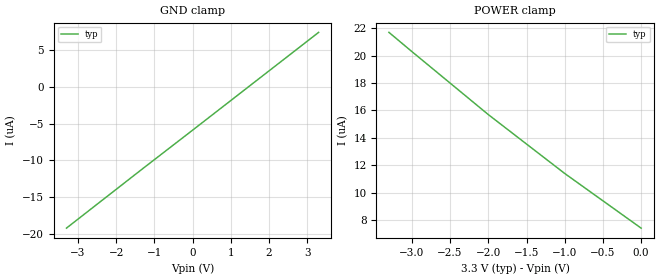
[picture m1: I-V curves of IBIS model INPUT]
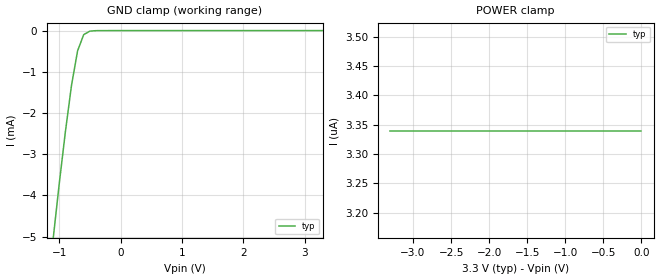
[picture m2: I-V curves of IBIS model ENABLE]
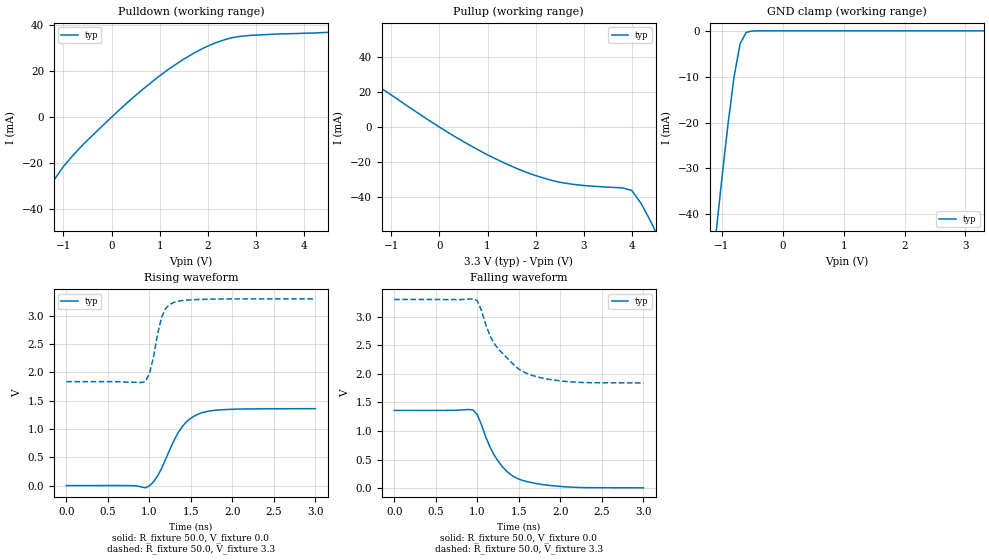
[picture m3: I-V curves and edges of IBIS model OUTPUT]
|   Texas Instruments Incorporated
|   Data Transmissions Products
|   IBIS Model for SN65LVDS348
|   16D SOIC Package
[IBIS Ver]   3.2
[Comment char]   |_char
[File name]   lvds348.ibs
[File Rev]   1.0
[Date]   23Aug01
[Source]   File originated at Texas Instruments Incorporated.
   Data Transmission Products Group. All data based on
   Bench Measurements.
[Notes]
[Disclaimer]
(C) Copyright Texas Instruments Incorporated 2001
   All rights reserved
  Texas Instruments Incorporated hereby grants the user of this IBIS
model a non-exclusive, nontransferable license to use this IBIS model
under the following terms.  Before using this IBIS model, the user
should read this license.  If the user does not accept these terms,
the IBIS model should be returned to Texas Instruments within 30 days.
  The user is granted this license only to use the IBIS model and
is not granted rights to sell, load, rent, lease or license the IBIS
model in whole or in part, or in modified form to anyone other than
user.  User may modify the IBIS model to suit its specific applications
but rights to derivative works and such modifications shall belong to
Texas Instruments.
  This IBIS model is provided on an "AS IS" basis and Texas Instruments
makes absolutely no warranty with respect to the information contained
herein.  TEXAS INSTRUMENTS DISCLAIMS AND CUSTOMER WAIVES ALL WARRANTIES,
EXPRESS OR IMPLIED, INCLUDING WARRANTIES OF MERCHANTABILITY OR FITNESS
FOR A PARTICULAR PURPOSE. The entire risk as to quality and performance
is with the Customer. ACCORDINGLY, IN NO EVENT SHALL THE COMPANY BE LIABLE
FOR ANY DAMAGES, WHETHER IN CONTRACT OR TORT,INCLUDING ANY LOST PROFITS
OR OTHER INCIDENTAL, CONSEQUENTIAL, EXEMPLARY, OR PUNITIVE DAMAGES ARISING
OUT OF THE USE OR APPLICATION OF THE IBIS model provided in this package.
Further, Texas Instruments reserves the right to discontinue or make changes
without notice to any product herein to improve reliability, function, or
design. Texas Instruments does not convey any license under patent rights
or any other intellectual property rights, including those of third parties.
Contact Texas Instruments at ATTN:DATA TRANSMISSIONS
[Copyright]   Copyright 2001, Texas Instruments, All Rights Reserved
[Component]   SN65LVDS348D
[Manufacturer]  Texas Instruments Incorporated
[Package]
|   typ   min   max
R_pkg   0.035   0.030   0.040
L_pkg   2.181nH   1.231nH   3.257nH
C_pkg   0.322pF   0.163pF   0.546pF
[Pin]   signal_name   model_name   R_pin   L_pin   C_pin
1   RIN1-   INPUT   0.040   3.251n   0.546p
2   RIN1+   INPUT   0.039   2.561n   0.393p
3   RIN2+   INPUT   0.030   1.681n   0.186p
4   RIN2-   INPUT   0.030   1.231n   0.163p
5   RIN3-   INPUT   0.030   1.231n   0.163p
6   RIN3+   INPUT   0.030   1.681n   0.186p
7   RIN4+   INPUT   0.039   2.564n   0.393p
8   RIN4-   INPUT   0.040   3.257n   0.545p
9   /EN   ENABLE   0.040   3.247n   0.546p
10   ROUT4   OUTPUT   0.039   2.558n   0.394p
11   ROUT3   OUTPUT   0.030   1.681n   0.187p
12   GND   GND   0.030   1.231n   0.163p
13   VCC   POWER   0.030   1.231n   0.163p
14   ROUT2   OUTPUT   0.030   1.681n   0.187p
15   ROUT1   OUTPUT   0.039   2.558n   0.394p
16   EN   ENABLE   0.040   3.246n   0.546p
[Diff_pin]   inv_pin   vdiff   tdelay_typ   tdelay_min   tdelay_max
| The 'xA' pin is Diff_pin and the 'xB' pin is the inv_pin
2   1   50mV   0 0 0   | Vth  +/-50mV
6   7   50mV   0 0 0
10   9   50mV   0 0 0
14   15   50mV   0 0 0
| Models and submodels in the file (3): INPUT (Input), ENABLE (Input), OUTPUT (3-state)
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|   Receiver Input Model
[Model]   INPUT
Model_type   Input
|Signals   RIN1-,RIN1+,RIN2+,RIN2-,RIN3-,RIN3+,RIN4+,RIN4-
Vinh = 2.0
Vinl = 0.8
|   typ   min   max
C_comp   1.0pF   NA   NA
|   typ   min   max
[Temperature Range]   25.0   NA   NA
[Voltage range]   3.3V   3.0V   3.6V
[GND_clamp]
|   Voltage   I(typ)   I(min)   I(max)
-3.3V     -19.2uA    NA         NA
-1.3V     -11.1uA    NA         NA
0V        -5.89uA    NA         NA
1.3V      -651nA     NA         NA
3.3V      7.41uA     NA         NA
[Power_clamp]
| Note that the[POWER_clamp]voltage table is referenced to Vcc
| and is calculated using Vtable=Vcc - Vmeasured.
|   Voltage   I(typ)   I(min)   I(max)
-3.3V     21.7uA     NA         NA
-3V       20.3uA     NA         NA
-2V       15.7uA     NA         NA
-1V       11.4uA     NA         NA
0V        7.41uA     NA         NA
|   Receiver Enable Model
[Model]   ENABLE
Model_type   Input
|Signals   /EN, EN
Vinh = 2.0
Vinl = 0.8
|   typ   min   max
C_comp   1.0pF   NA   NA
|   typ   min   max
[Temperature Range]   25.0   NA   NA
[Voltage range]   3.3V   3.0V   3.6V
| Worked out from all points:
|   GND clamp passes 1 mA (typ) near -0.76 V on its own axis
[GND_clamp]
|   Voltage   I(typ)   I(min)   I(max)
-3.3V     -43.1mA    NA         NA
-1.1V     -5.08mA    NA         NA
-1V       -3.73mA    NA         NA
-900mV    -2.47mA    NA         NA
-800mV    -1.34mA    NA         NA
-700mV    -493uA     NA         NA
-600mV    -98.5uA    NA         NA
-500mV    -13.3uA    NA         NA
3.3V      3.34pA     NA         NA
[Power_clamp]
| Note that the[POWER_clamp]voltage table is referenced to Vcc
| and is calculated using Vtable=Vcc - Vmeasured.
|   Voltage   I(typ)   I(min)   I(max)
-3.3V     3.34uA     NA         NA
-2.7V     3.34uA     NA         NA
-2V       3.34uA     NA         NA
-800mV    3.34uA     NA         NA
0V        3.34uA     NA         NA
|   Receiver Output Model
[Model]   OUTPUT
Model_type   3-state
|Signals   ROUT1,ROUT2,ROUT3,ROUT4
Vmeas = 1.5V   |Reference voltage for timing measurements
Cref = 8pF   |Timing specification test load capacitance value
Vref = 0   |Timing specification test load voltage; GND
| variable   typ   min   max
C_comp   1.0pF   NA   NA
|   typ   min   max
[Temperature Range]   25.0   NA   NA
[Voltage range]   3.3V   3.0V   3.6V
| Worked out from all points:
|   slope of the pulldown table from 0 to 0.495 V, typ, clamps not added: 52.7 ohm
|   slope of the pullup table from 0 to 0.495 V, typ, clamps not added: 60.3 ohm
|   GND clamp passes 1 mA (typ) near -0.63 V on its own axis
|   rising waveform, R_fixture 50.0, V_fixture 0.0: 20-80 % time 287ps typ, NA min, NA max; typ from 0.001 V to 1.36 V
|   falling waveform, R_fixture 50.0, V_fixture 0.0: 20-80 % time 315ps typ, NA min, NA max; typ from 1.36 V to 0.004 V
|   rising waveform, R_fixture 50.0, V_fixture 3.3: 20-80 % time 131ps typ, NA min, NA max; typ from 1.84 V to 3.3 V
|   falling waveform, R_fixture 50.0, V_fixture 3.3: 20-80 % time 389ps typ, NA min, NA max; typ from 3.3 V to 1.84 V
[Pulldown]
|   Voltage   I(typ)   I(min)   I(max)
-3.3V     -150mA     NA         NA
-1.6V     -47.9mA    NA         NA
-1.2V     -27.5mA    NA         NA
-1V       -21.5mA    NA         NA
-600mV    -12.1mA    NA         NA
200mV     3.91mA     NA         NA
900mV     16.4mA     NA         NA
1.5V      25.3mA     NA         NA
2.1V      31.9mA     NA         NA
2.5V      34.6mA     NA         NA
2.9V      35.7mA     NA         NA
6.6V      39.1mA     NA         NA
[Pullup]
|   Voltage   I(typ)   I(min)   I(max)
| Note that the[Pullup]voltage table is referenced to Vcc
| and is calculated using Vtable=Vcc - Vmeasured.
-3.3V     61mA       NA         NA
-3.1V     57.2mA     NA         NA
-3V       55.4mA     NA         NA
100mV     -1.72mA    NA         NA
900mV     -14.4mA    NA         NA
1.6V      -23.5mA    NA         NA
2.5V      -31.4mA    NA         NA
4V        -36.1mA    NA         NA
4.2V      -43.8mA    NA         NA
4.4V      -54.1mA    NA         NA
4.6V      -65.3mA    NA         NA
6.6V      -187mA     NA         NA
| Output in High Impedance (off)
[GND_clamp]
|   Voltage   I(typ)   I(min)   I(max)
-3.3V     -347mA     NA         NA
-1.1V     -44.7mA    NA         NA
-1V       -32.3mA    NA         NA
-900mV    -20.5mA    NA         NA
-800mV    -10.1mA    NA         NA
-700mV    -2.82mA    NA         NA
-600mV    -350uA     NA         NA
-500mV    -29.4uA    NA         NA
-400mV    -1.91uA    NA         NA
3.3V      426pA      NA         NA
[POWER_clamp]
|   Voltage   I(typ)   I(min)   I(max)
| Note that the [POWER_clamp] voltage table is referenced to Vcc
| and is calculated using Vtable = Vcc - Vmeasured.
| Outputs in Tri-state.
-3.3V     0A         NA         NA
0V        0A         NA         NA
[Ramp]
|   typ   min   max
dV/dt_r   0.815V/389ps   NA   NA
dV/dt_f   0.880V/285ps   NA   NA
R_load = 50
[Rising Waveform]
R_fixture = 50.0
V_fixture = 0.0
C_fixture = 0p
L_fixture = 0n
|   V(typ)   V(min)   V(max)
0s        1mV        NA         NA
950ps     -39mV      NA         NA
1ns       -5mV       NA         NA
1.1ns     171mV      NA         NA
1.3ns     807mV      NA         NA
1.4ns     1.051V     NA         NA
1.5ns     1.192V     NA         NA
1.65ns    1.295V     NA         NA
2.05ns    1.351V     NA         NA
3ns       1.359V     NA         NA
[Falling Waveform]
R_fixture = 50.0
V_fixture = 0.0
C_fixture = 0p
L_fixture = 0n
|   V(typ)   V(min)   V(max)
0s        1.359V     NA         NA
950ps     1.365V     NA         NA
1ns       1.285V     NA         NA
1.15ns    728mV      NA         NA
1.25ns    474mV      NA         NA
1.4ns     239mV      NA         NA
1.55ns    132mV      NA         NA
1.8ns     59mV       NA         NA
2.05ns    23mV       NA         NA
3ns       4mV        NA         NA
[Rising Waveform]
R_fixture = 50.0
V_fixture = 3.3
C_fixture = 0p
L_fixture = 0n
|   V(typ)   V(min)   V(max)
0s        1.836V     NA         NA
950ps     1.834V     NA         NA
1ns       1.971V     NA         NA
1.05ns    2.27V      NA         NA
1.1ns     2.682V     NA         NA
1.15ns    2.984V     NA         NA
1.2ns     3.135V     NA         NA
1.3ns     3.238V     NA         NA
1.7ns     3.292V     NA         NA
3ns       3.298V     NA         NA
[Falling Waveform]
R_fixture = 50.0
V_fixture = 3.3
C_fixture = 0p
L_fixture = 0n
|   V(typ)   V(min)   V(max)
0s        3.299V     NA         NA
950ps     3.311V     NA         NA
1ns       3.279V     NA         NA
1.05ns    3.109V     NA         NA
1.15ns    2.674V     NA         NA
1.2ns     2.537V     NA         NA
1.45ns    2.144V     NA         NA
1.65ns    1.977V     NA         NA
2.1ns     1.862V     NA         NA
3ns       1.84V      NA         NA
